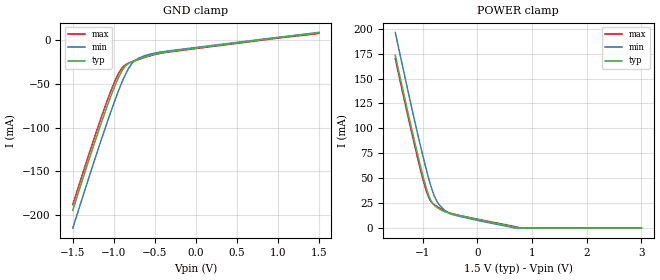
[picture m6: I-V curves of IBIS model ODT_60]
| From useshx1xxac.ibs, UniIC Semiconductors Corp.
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|   Model ODT_60
[Model]  ODT_60
Model_type   Input
Polarity   Non-Inverting
Vinl =   0.600000V
Vinh =   0.900000V
C_comp   1.3900pF   1.3640pF   1.5600pF
[Temperature Range]   25.0000   95.0000   0.0
[Voltage Range]   1.5000V   1.4000V   1.6000V
[GND_clamp]
|Voltage   I(typ)   I(min)   I(max)
-1.5V     -194.4mA   -214.8mA   -188mA
-1.18V    -102.1mA   -121.5mA   -95.53mA
-1.06V    -70.01mA   -88.2mA    -63.88mA
-980mV    -50.55mA   -67.1mA    -45.17mA
-940mV    -41.97mA   -57.14mA   -37.41mA
-900mV    -34.78mA   -47.78mA   -31.58mA
-860mV    -29.58mA   -39.3mA    -28.07mA
-780mV    -24.53mA   -26.63mA   -24.59mA
-740mV    -23.04mA   -22.95mA   -23.25mA
-620mV    -19.15mA   -17.55mA   -19.51mA
-420mV    -14.26mA   -13.3mA    -14.69mA
1.5V      8.718mA    9.062mA    7.852mA
[POWER_clamp]
|Voltage   I(typ)   I(min)   I(max)
-1.5V     173.4mA    196.3mA    170mA
-1.12V    80.51mA    101.5mA    76.96mA
-1V       53.63mA    73.55mA    50.23mA
-920mV    37.89mA    56.11mA    35.24mA
-880mV    31.5mA     48.01mA    29.81mA
-840mV    26.75mA    40.58mA    26.32mA
-760mV    21.7mA     29.02mA    22.53mA
-680mV    18.79mA    22.41mA    19.91mA
-580mV    16.2mA     17.18mA    17.11mA
-320mV    12.49mA    11.79mA    12.66mA
752.8mV   0A         NA         NA
3V        0A         0A         0A
